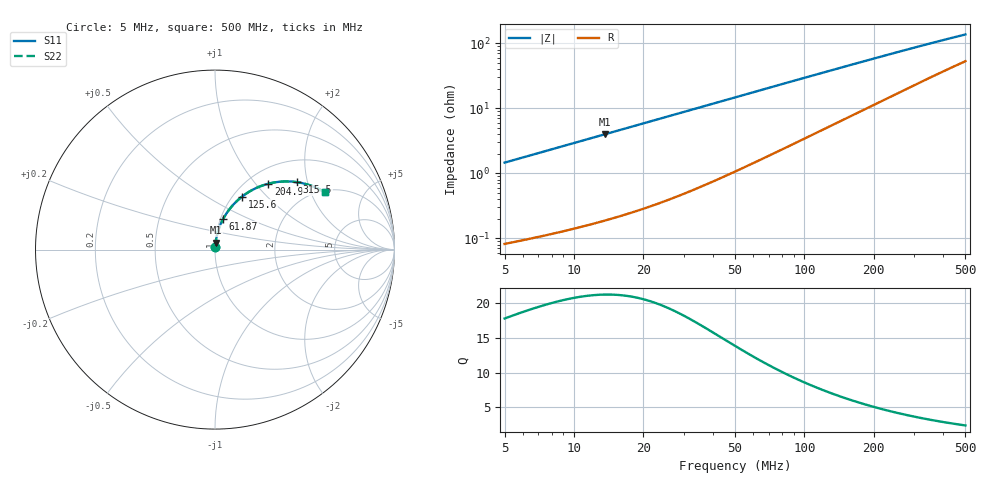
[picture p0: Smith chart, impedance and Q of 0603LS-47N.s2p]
# MHz S MA R 50
!Freq  MagS11  AngS11  MagS21  AngS21  MagS12  AngS12  MagS22  AngS22
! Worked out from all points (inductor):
!   801 points, 5 MHz to 500 MHz, reference 50 ohm
!   read as one part in series: L = 46.3 nH near 5.116 MHz
!   highest Q = 21.2 at 13.61 MHz (marker M1), where L = 46.4 nH
!   S11 on the Smith chart (normalised r, x): 5 MHz: 1.00, +0.03; 61.87 MHz: 1.03, +0.36; 125.6 MHz: 1.10, +0.73; 204.9 MHz: 1.24, +1.17; 315.5 MHz: 1.49, +1.73; 500 MHz: 2.06, +2.52
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5  0.01454 86.0  0.9991 -0.8  0.9991 -0.8  0.01454 86.0
6.744814  0.01962 85.9  0.9988 -1.1  0.9988 -1.1  0.01962 85.9
8.63913  0.02512 85.7  0.9984 -1.4  0.9984 -1.4  0.02512 85.7
10.93881  0.03181 85.4  0.998 -1.8  0.998 -1.8  0.03181 85.4
13.61351  0.0396 85.0  0.9974 -2.3  0.9974 -2.3  0.0396 85.0
17.23733  0.05015 84.4  0.9964 -2.9  0.9964 -2.9  0.05015 84.4
21.45211  0.06242 83.6  0.995 -3.6  0.995 -3.6  0.06242 83.6
26.39186  0.07676 82.6  0.993 -4.4  0.993 -4.4  0.07676 82.6
31.91317  0.09271 81.5  0.9905 -5.3  0.9905 -5.3  0.09271 81.5
45.3388  0.1309 78.6  0.9825 -7.5  0.9825 -7.5  0.1309 78.6
61.86856  0.1765 75.1  0.9698 -10.1  0.9698 -10.1  0.1765 75.1
73.95542  0.2086 72.7  0.9587 -12.0  0.9587 -12.0  0.2086 72.7
87.89618  0.2441 69.9  0.9443 -14.0  0.9443 -14.0  0.2441 69.9
105.6745  0.2868 66.5  0.9241 -16.5  0.9241 -16.5  0.2868 66.5
125.5943  0.3312 63.0  0.8994 -19.2  0.8994 -19.2  0.3312 63.0
170.4002  0.4174 55.8  0.8398 -24.3  0.8398 -24.3  0.4174 55.8
204.8661  0.4719 51.0  0.7933 -27.6  0.7933 -27.6  0.4719 51.0
253.4954  0.5336 45.3  0.7307 -31.3  0.7307 -31.3  0.5336 45.3
315.4787  0.5923 39.3  0.6592 -34.7  0.6592 -34.7  0.5923 39.3
336.1012  0.608 37.6  0.6378 -35.6  0.6378 -35.6  0.608 37.6
418.2828  0.6566 32.0  0.5634 -38.1  0.5634 -38.1  0.6566 32.0
500  0.6894 27.7  0.5049 -39.5  0.5049 -39.5  0.6894 27.7
